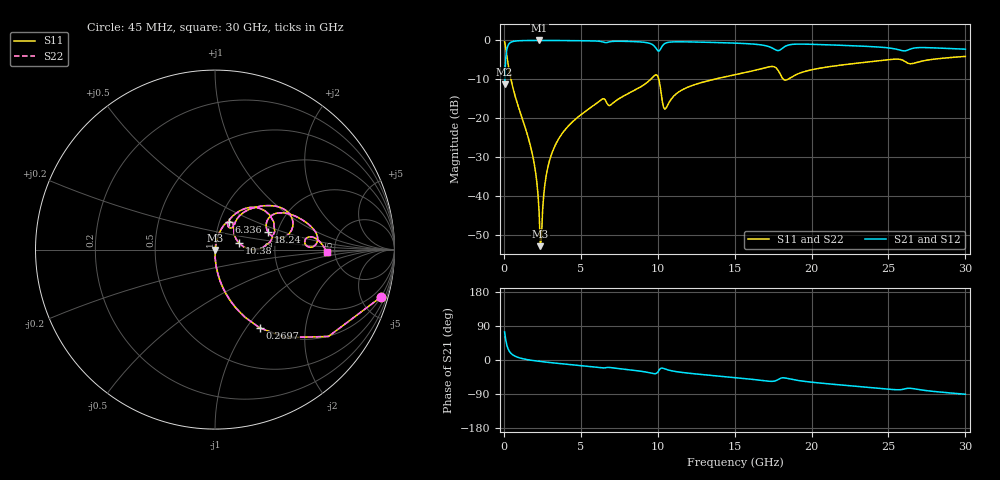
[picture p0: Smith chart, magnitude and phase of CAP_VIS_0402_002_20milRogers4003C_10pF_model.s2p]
! S-parameter model data by Modelithics Inc.  support@modelithics.com  813-866-6335  Tampa FL USA
! S-Parameter data specifications:
! Substrate: 20-mil Rogers 4003C, substrate thickness, H=0.508mm, Dielectric constant, Er=3.75
! PCB Mounting Pad Footprint: Pad width, PadW=0.50mm , Pad length, PadL=0.50mm , Pad gap, PadG (edge-to-edge)=0.40mm , Reference planes=1.4mm apart
! Created Wed Nov 18 12:50:46 2015
# hz S ma R 50
! 2 Port Network Data from SP1.SP block
! freq  magS11  angS11  magS21  angS21  magS12  angS12  magS22  angS22
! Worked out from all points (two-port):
!   401 points, 45 MHz to 30 GHz, reference 50 ohm
!   highest |S21| = -0.01 dB at 2.292 GHz (marker M1); lowest = -11.3 dB at 45 MHz (marker M2)
!   |S21| within 3 dB of the highest: 166.2 MHz to end of sweep
!   lowest |S11| = -52.8 dB at 2.367 GHz (marker M3), VSWR 1.00, Z = 50.1 - j0.178 ohm
!   |S11| at or under -10 dB: 458.2 MHz to 9.537 GHz (9.079 GHz wide, 182 % of centre); 10.07 GHz to 13.65 GHz (3.575 GHz wide, 30.2 % of centre); 18.18 GHz to 18.45 GHz (266.1 MHz wide, 1.45 % of centre)
!   |S22| runs from -52.8 to -0.3 dB; largest |S21 - S12| = 0
!   S11 on the Smith chart (normalised r, x): 45 MHz: 0.99, -7.00; 269.7 MHz: 0.99, -1.15; 6.336 GHz: 1.11, +0.36; 10.38 GHz: 1.30, +0.10; 18.24 GHz: 1.78, +0.39; 30 GHz: 4.30, -0.18
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4.5e7  0.9618 -16.0  0.2736 74.0  0.2736 74.0  0.9618 -16.0
2.696625e8  0.5011 -60.3  0.8649 29.6  0.8649 29.6  0.5011 -60.3
6.441e8  0.2222 -78.0  0.9742 11.8  0.9742 11.8  0.2222 -78.0
1.8423e9  0.03526 -88.8  0.9979 -1.1  0.9979 -1.1  0.03526 -88.8
2.066962e9  0.01975 -88.1  0.9983 -2.3  0.9983 -2.3  0.01975 -88.1
2.291625e9  0.006143 -78.9  0.9984 -3.5  0.9984 -3.5  0.006143 -78.9
2.366512e9  0.002294 -50.6  0.9984 -3.9  0.9984 -3.9  0.002294 -50.6
2.516288e9  0.006701 71.4  0.9983 -4.6  0.9983 -4.6  0.006701 71.4
2.815838e9  0.02169 79.5  0.998 -6.0  0.998 -6.0  0.02169 79.5
3.190275e9  0.03889 79.7  0.9973 -7.6  0.9973 -7.6  0.03889 79.7
5.062462e9  0.1135 73.5  0.9905 -15.0  0.9905 -15.0  0.1135 73.5
6.33555e9  0.1737 63.2  0.9659 -20.6  0.9659 -20.6  0.1737 63.2
6.93465e9  0.1483 60.5  0.9646 -20.0  0.9646 -20.0  0.1483 60.5
9.555712e9  0.3188 47.6  0.9045 -34.4  0.9045 -34.4  0.3188 47.6
1.007992e10  0.3119 8.0  0.7288 -27.3  0.7288 -27.3  0.3119 8.0
1.037948e10  0.1385 15.0  0.8859 -22.2  0.8859 -22.2  0.1385 15.0
1.50225e10  0.3631 42.2  0.9229 -46.5  0.9229 -46.5  0.3631 42.2
1.74189e10  0.4632 22.7  0.8023 -56.4  0.8023 -56.4  0.4632 22.7
1.824266e10  0.311 18.4  0.8299 -47.2  0.8299 -47.2  0.311 18.4
2.003996e10  0.4214 29.1  0.8906 -58.7  0.8906 -58.7  0.4214 29.1
2.505742e10  0.5669 10.4  0.7988 -77.2  0.7988 -77.2  0.5669 10.4
3e10  0.6233 -1.1  0.7718 -90.3  0.7718 -90.3  0.6233 -1.1
